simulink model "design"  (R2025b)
settings: Solver=VariableStepAuto  StartTime=0.0  StopTime=10.0  RelTol=1e-3
InitFcn:
  | SSR=8;
undefined symbols (not defined in the file or in its folder): code, Evaluation, KC705, Kintex, netlist, Platform, xc7k325tffg900
libraries: hlsBasic x6, design_lib x2, vmcUtilities x1

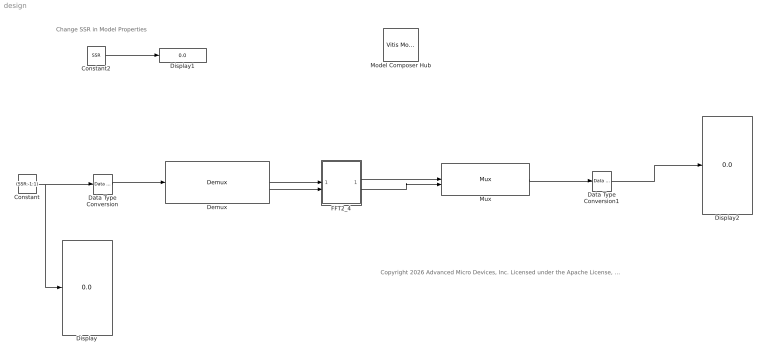
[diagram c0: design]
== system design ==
  note: Change SSR in Model Properties
  note: Copyright 2026 Advanced Micro Devices, Inc. Licensed under the Apache License, Version 2.0 (the "License"); you may not use this file except in compliance with the License. You may obtain a copy of the License at http://www.apache.org/licenses/LICENSE-2.0 Unless required by applicable law or agreed to in writing, software distributed under the License is distributed on an "AS IS" BASIS, WITHOUT WARRANTIES OR CONDITIONS OF ANY KIND, either express or implied. See the License for the specific language governing permissions and limitations under the License.
  Constant : Constant  Value=(SSR:-1:1)  SampleTime=1
  Constant2 : Constant  Value=SSR  VectorParams1D=off  SampleTime=1
  Data Type Conversion : hlsBasic/Data Type Conversion  OutDataType=fixed  TypeExp=''  Signedness=Signed  WordLength=32  FractionalLength=16  RoundingMode=Truncation to minus infinity  OverflowMode=Wrap around
  Data Type Conversion1 : hlsBasic/Data Type Conversion  OutDataType=double  TypeExp=''  Signedness=Signed  WordLength=16  FractionalLength=0  RoundingMode=Truncation to minus infinity  OverflowMode=Wrap around
  Demux : design_lib/Demux  LibraryFunction=Demux  IncludeFiles={'template_design.h'}  SourceFiles={}  IncludeDirectories={}  TemplateParams={'int NUMOFELEMENTS'; 'int W'; 'int I'}  FunctionParamTypes={xmcDataType('void'); xmcDataType('ap_fixed<W, I>'); xmcDataType('ap_fixed<W, I>'); xmcDataType('ap_fixed<W, I>')}  FunctionParamPassbys={0.000000000000000000e+00; 0.000000000000000000e+00; 0.000000000000000000e+00; 0.000000000000000000e+00}  FunctionParamDimensions={'1'; '[NUMOFELEMENTS]'; '[NUMOFELEMENTS / 2]'; '[NUMOFELEMENTS / 2]'}  FunctionParamNames={'return'; 'vector_in'; 'vector_out0'; 'vector_out1'}  FunctionParamDir={0.000000000000000000e+00; 1.000000000000000000e+00; 2.000000000000000000e+00; 2.000000000000000000e+00}  FunctionParamSupportsStreaming={false; false; false; false}  BufferDepth={'0'}  FunctionParamValues={'0'; '0'; '0'; '0'}  ThroughputFactors={''}
  Display : Display
  Display1 : Display
  Display2 : Display
  FFT2_4 : Subsystem
  Model Composer Hub : vmcUtilities/Vitis Model Composer Hub  Tag=genX  CodeGeneration=off  SubsystemName=Subsystem  StartColumn=1  NumberOfColumns=1  TargetDirectory=./code  exportDesign=off  analyzeDesign=off  validateDesignOnHw=off  ExportType=IP Catalog  IpVendor=xilinx.com  IpLibrary=hls  IpVersion=1.0  IpHWLanguage=Verilog  AieCompilerOptions={}  AieSimulatorOptions={}  CreateTestbench=off  TestbenchStackSize=10  RunRtlSim=off  RunCSim=off  RunAieSim=off  AieSimTimeout=50000  RunAieSimProfiling=off  LaunchVitisAnalyzer=off  PlotOutput=off  RunX86Sim=on  X86SimTimeout=10  GenHwImage=off  GenLibadfXo=off  GenHwValidationCode=off  PlatformType=Not Specified  HwSystemType=Baremetal  HwValidationTarget=hw  ProjDevice=Kintex-7 KC705 Evaluation Platform (xc7k325tffg900-2)  ProjDevicePart=xc7k325tffg900-2  SamplePeriod=-1  ClockFrequency=200  DataPathParallelism=1  xilinxfamily=Kintex7  part=xc7k325t  speed=-3  package=fbg676  directory=./netlist  testbench=off  incr_netlist=off  synthesis_tool=Vivado  clock_wrapper=Clock Enables  dbl_ovrd=According to Block Masks  dcm_input_clock_period=10  sysclk_period=10  simulink_period=1  eval_field=0  LogFileName=''  NThreads=4
  Mux : design_lib/Mux  LibraryFunction=Mux  IncludeFiles={'template_design.h'}  SourceFiles={}  IncludeDirectories={}  TemplateParams={'int NUMOFELEMENTS'; 'int W'; 'int I'}  FunctionParamTypes={xmcDataType('void'); xmcDataType('ap_fixed<W, I>'); xmcDataType('ap_fixed<W, I>'); xmcDataType('ap_fixed<W, I>')}  FunctionParamPassbys={0.000000000000000000e+00; 0.000000000000000000e+00; 0.000000000000000000e+00; 0.000000000000000000e+00}  FunctionParamDimensions={'1'; '[NUMOFELEMENTS]'; '[NUMOFELEMENTS]'; '[NUMOFELEMENTS * 2]'}  FunctionParamNames={'return'; 'vector_in0'; 'vector_in1'; 'vector_out'}  FunctionParamDir={0.000000000000000000e+00; 1.000000000000000000e+00; 1.000000000000000000e+00; 2.000000000000000000e+00}  FunctionParamSupportsStreaming={false; false; false; false}  BufferDepth={'0'}  FunctionParamValues={'0'; '0'; '0'; '0'}  ThroughputFactors={''}
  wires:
  Constant/1 -> Display/1, Data Type Conversion/1
  Data Type Conversion/1 -> Demux/1
  Mux/1 -> Data Type Conversion1/1
  FFT2_4/1(O0) -> Mux/1
  FFT2_4/2(O1) -> Mux/2
  Demux/1 -> FFT2_4/1(I0)
  Demux/2 -> FFT2_4/2(I1)
  Constant2/1 -> Display1/1
  Data Type Conversion1/1 -> Display2/1

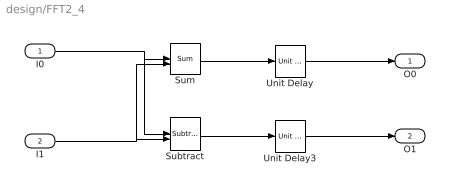
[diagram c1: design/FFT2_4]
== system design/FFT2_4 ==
  I0 : Inport
  I1 : Inport  Port=2
  Subtract : hlsBasic/Subtract
  Sum : hlsBasic/Sum
  Unit Delay : hlsBasic/Unit Delay  InitialCondition=0
  Unit Delay3 : hlsBasic/Unit Delay  InitialCondition=0
  O0 : Outport
  O1 : Outport  Port=2
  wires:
  Sum/1 -> Unit Delay/1
  Unit Delay/1 -> O0/1
  Subtract/1 -> Unit Delay3/1
  Unit Delay3/1 -> O1/1
  I0/1 -> Subtract/1, Sum/1
  I1/1 -> Subtract/2, Sum/2
